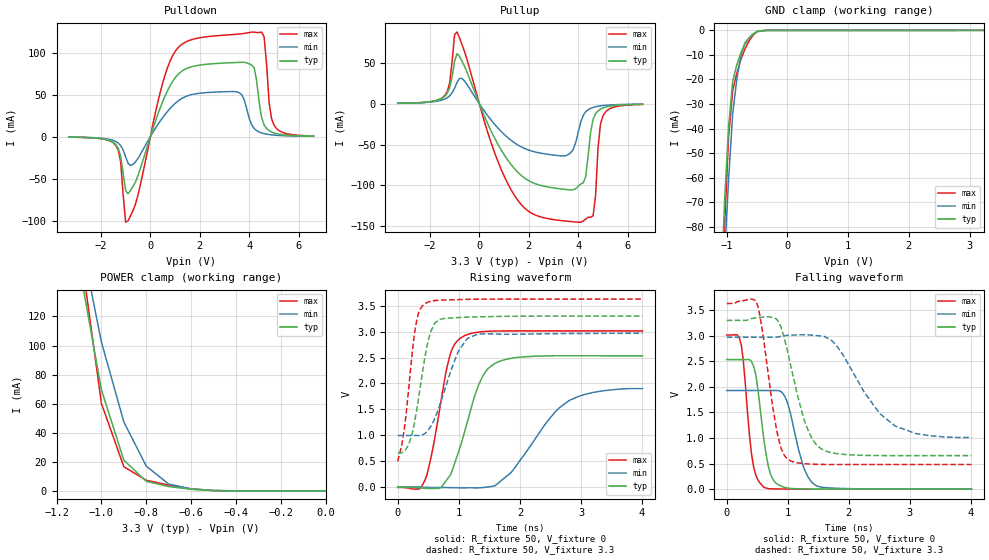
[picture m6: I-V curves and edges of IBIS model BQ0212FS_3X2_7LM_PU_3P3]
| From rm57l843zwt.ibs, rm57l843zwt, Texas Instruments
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|   Model Cell FS_3X2_7LM_PU_3P3
|BQ0212FS_3X2_7LM_PU_3P3
[Model]   BQ0212FS_3X2_7LM_PU_3P3
Model_type   I/O
Polarity   Non-Inverting
Enable   Active-Low
Vinl =  1.25
Vinh =  1.65
Cref =  15.0001pF
Rref =  101.0000M
Vref =  0V
Vmeas =  1.65
C_comp   1.2p   1.2p   1.2p
[Model Spec]
Vinl   1.25   1.12   1.38
Vinh   1.65   1.45   1.75
[Temperature Range]   25   155   -40
[Voltage Range]   3.3   2.97   3.63
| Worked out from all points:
|   slope of the pulldown table from 0 to 0.495 V, typ, clamps not added: 11.9 ohm
|   slope of the pullup table from 0 to 0.495 V, typ, clamps not added: 14.3 ohm
|   GND clamp passes 1 mA (typ) near -0.53 V on its own axis
|   POWER clamp passes 1 mA (typ) near -0.59 V on its own axis
|   rising waveform, R_fixture 50, V_fixture 0: 20-80 % time 399ps typ, 715ps min, 277ps max; typ from 0 V to 2.53 V
|   rising waveform, R_fixture 50, V_fixture 3.3: 20-80 % time 225ps typ, 347ps min, 172ps max; typ from 0.657 V to 3.3 V
|   falling waveform, R_fixture 50, V_fixture 0: 20-80 % time 170ps typ, 243ps min, 138ps max; typ from 2.53 V to 0 V
|   falling waveform, R_fixture 50, V_fixture 3.3: 20-80 % time 342ps typ, 655ps min, 230ps max; typ from 3.3 V to 0.657 V
[POWER_clamp]
|   voltage   I(typ)   I(min)   I(max)
-3.3V     2.375A     2.63A      3.153A
-1.1V     156mA      180.2mA    173.4mA
-1.067V   127.2mA    154.3mA    135.7mA
-1.033V   98.42mA    128.4mA    97.93mA
-1V       69.62mA    102.5mA    60.21mA
-900mV    21.14mA    47.42mA    16.63mA
-800mV    6.589mA    17.01mA    7.329mA
-700mV    3.011mA    4.694mA    4.008mA
-600mV    1.098mA    1.411mA    1.442mA
-500mV    196.6uA    363.8uA    217.1uA
0V        311pA      5.944nA    271.9pA
[Pulldown]
|   voltage   I(typ)   I(min)   I(max)
-3.3V     -554.3uA   -511.5uA   -526.2uA
-1.4V     -9.291mA   -5.703mA   -10.34mA
-1.2V     -23.68mA   -10.64mA   -30.19mA
-1V       -64.35mA   -24mA      -101.9mA
-600mV    -53.61mA   -29.92mA   -79.98mA
1V        70.16mA    39.6mA     101.5mA
3.5V      88.44mA    53.42mA    122.1mA
4.2V      81.93mA    9.711mA    124.7mA
4.6V      13.96mA    3.646mA    118.8mA
4.8V      7.183mA    2.57mA     41.14mA
5V        4.453mA    1.905mA    13.75mA
6.6V      621.1uA    479.2uA    840.9uA
[Pullup]
|   voltage   I(typ)   I(min)   I(max)
-3.3V     614.6uA    591.9uA    551.1uA
-1.4V     9.028mA    5.738mA    10.01mA
-900mV    61.32mA    26.24mA    87.8mA
1.4V      -78.76mA   -47.33mA   -111.2mA
3.5V      -105mA     -63.56mA   -143.7mA
4.1V      -98.29mA   -22.39mA   -145.1mA
4.3V      -89.13mA   -9.839mA   -141.1mA
4.6V      -19.02mA   -4.469mA   -137.2mA
4.7V      -12.15mA   -3.653mA   -112.5mA
4.8V      -8.616mA   -3.042mA   -53.65mA
5V        -5.089mA   -2.205mA   -14.76mA
6.6V      -663.5uA   -536.5uA   -825.6uA
[GND_clamp]
|   voltage   I(typ)   I(min)   I(max)
-3.3V     -1.947A    -1.623A    -3.254A
-1.1V     -112mA     -127mA     -135.8mA
-1.033V   -69.61mA   -91.63mA   -80.19mA
-966.7mV  -39.23mA   -60.62mA   -43.12mA
-900mV    -20.87mA   -34.02mA   -24.53mA
-833.3mV  -14.27mA   -20.12mA   -17.62mA
-766.7mV  -9.205mA   -10.52mA   -12.03mA
-700mV    -5.683mA   -5.213mA   -7.735mA
-566.7mV  -1.585mA   -1.582mA   -2.087mA
-500mV    -421.6uA   -595.6uA   -492.4uA
-300mV    -20.33uA   -17.44uA   -33.22uA
3.233V    -1.13uA    6.924uA    -9.303uA
[Ramp]
| variable   typ   min   max
dV/dt_f   1.631812/0.3488821n   1.217121/0.6771253n   1.942036/0.2339415n
dV/dt_r   1.539696/0.4016612n   1.169959/0.7432805n   1.834863/0.2803582n
R_load = 50
[Rising Waveform]
R_fixture = 50
V_fixture = 0
V_fixture_min = 0
V_fixture_max = 0
|   time   V(typ)   V(min)   V(max)
0s        468.4uV    143.3uV    -9.614mV
340ps     -15.32mV   -146.5uV   -43.42mV
444ps     -26.77mV   -6.816mV   124.2mV
580ps     -30.9mV    -9.591mV   770mV
816ps     158mV      -13.15mV   2.361V
1.024ns   777.5mV    -18.12mV   2.874V
1.332ns   1.994V     -17.82mV   2.992V
1.592ns   2.387V     23.49mV    3.012V
2.812ns   2.535V     1.673V     3.014V
4.008ns   2.534V     1.9V       3.014V
[Rising Waveform]
R_fixture = 50
V_fixture = 3.3
V_fixture_min = 2.97
V_fixture_max = 3.63
|   time   V(typ)   V(min)   V(max)
0s        656.5mV    993.6mV    493.3mV
104ps     688.3mV    993.6mV    1.081V
204ps     901.8mV    993.7mV    2.203V
308ps     1.471V     992.3mV    3.204V
444ps     2.497V     1.03V      3.542V
544ps     3.013V     1.174V     3.589V
612ps     3.174V     1.34V      3.602V
972ps     3.272V     2.563V     3.619V
1.152ns   3.281V     2.876V     3.625V
4.008ns   3.3V       2.969V     3.63V
[Falling Waveform]
R_fixture = 50
V_fixture = 0
V_fixture_min = 0
V_fixture_max = 0
|   time   V(typ)   V(min)   V(max)
0s        2.534V     1.93V      3.014V
240ps     2.534V     1.93V      2.818V
408ps     2.494V     1.93V      674.9mV
476ps     2.239V     1.93V      277.3mV
612ps     942.4mV    1.93V      34.57mV
716ps     298.8mV    1.93V      7.616mV
944ps     37.15mV    1.829V     3.558mV
1.256ns   5.735mV    439.5mV    1.262mV
1.464ns   3.351mV    67.77mV    850.9uV
4.008ns   266.9uV    929.5uV    189uV
[Falling Waveform]
R_fixture = 50
V_fixture = 3.3
V_fixture_min = 2.97
V_fixture_max = 3.63
|   time   V(typ)   V(min)   V(max)
0s        3.3V       2.97V      3.63V
476ps     3.349V     2.97V      3.686V
580ps     3.363V     2.97V      3.133V
816ps     3.327V     2.972V     1.168V
892ps     3.162V     2.99V      793.3mV
1.024ns   2.544V     3.01V      567.9mV
1.28ns    1.315V     3.021V     497.3mV
1.592ns   757.4mV    2.99V      483.6mV
2.756ns   656.1mV    1.236V     482.8mV
4.008ns   656.9mV    1.011V     482.5mV
